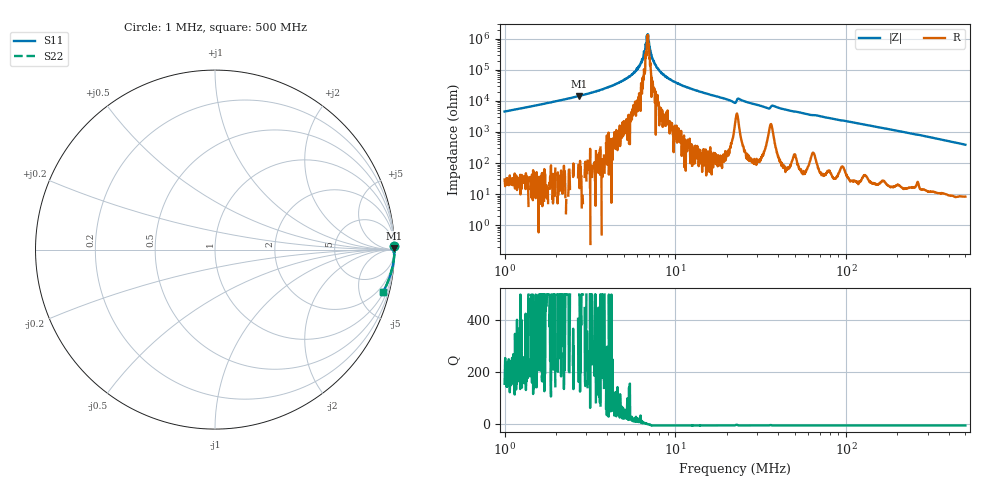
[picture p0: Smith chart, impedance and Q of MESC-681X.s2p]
!s-Parameter Generated by FASTRON Sdn. Bhd.
!FASTRON P/N : MESC-681X
!Keysight Technologies,E4991B,MY54100416,A.01.15
!Date: Fri Mar 27 12:52:29 2026
!Version  : Rev00 Fri Mar 27 12:52:29 2026
!Data & Calibration Information:
!PortZ  Port1:50+j0  Port2:50+j0
!When reading, reference impedance value at option line is always used.
!Remarks : This data is being provided solely for informational purposes.
!Freq	S11	S21	S12	S22
# Hz S dB R 50
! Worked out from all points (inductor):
!   1601 points, 1 MHz to 500 MHz, reference 50 ohm
!   read as one part in series: L = 713 uH near 1.032 MHz
!   highest Q = 942 at 2.745 MHz (marker M1), where L = 849 uH
!   self-resonance near 6.866 MHz
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1000000  -0.00 1.3  -33.22 -88.4  -33.22 -88.4  -0.00 1.3
2745255  -0.00 0.4  -43.31 -89.5  -43.31 -89.5  -0.00 0.4
2820919  -0.00 0.4  -43.64 -89.5  -43.64 -89.5  -0.00 0.4
4257919  -0.00 0.2  -49.74 -89.1  -49.74 -89.1  -0.00 0.2
5502118  -0.00 0.1  -56.67 -86.5  -56.67 -86.5  -0.00 0.1
5900561  -0.00 0.1  -59.62 -87.2  -59.62 -87.2  -0.00 0.1
6206152  -0.00 0.0  -63.32 -86.2  -63.32 -86.2  -0.00 0.0
6451950  -0.00 0.0  -67.45 -82.3  -67.45 -82.3  -0.00 0.0
6707483  -0.00 0.0  -76.90 -69.9  -76.90 -69.9  -0.00 0.0
6892354  -0.00 -0.0  -79.49 7.8  -79.49 7.8  -0.00 -0.0
7027516  -0.00 -0.0  -76.49 58.4  -76.49 58.4  -0.00 -0.0
7449115  -0.00 -0.0  -65.45 81.5  -65.45 81.5  -0.00 -0.0
7957584  -0.00 -0.1  -60.32 84.7  -60.32 84.7  -0.00 -0.1
8941017  -0.00 -0.1  -54.94 86.8  -54.94 86.8  -0.00 -0.1
1.094217e7  -0.00 -0.2  -50.07 89.3  -50.07 89.3  -0.00 -0.2
2.236068e7  -0.02 -0.6  -38.74 77.5  -38.74 77.5  -0.02 -0.6
2.37944e7  -0.01 -0.5  -41.17 83.5  -41.17 83.5  -0.01 -0.5
3.45472e7  -0.01 -1.0  -35.39 83.8  -35.39 83.8  -0.01 -1.0
3.762909e7  -0.01 -0.8  -36.82 83.3  -36.82 83.3  -0.01 -0.8
6.307767e7  -0.02 -1.6  -30.93 85.3  -30.93 85.3  -0.02 -1.6
1.77937e8  -0.04 -4.6  -21.88 84.5  -21.88 84.5  -0.04 -4.6
5e8  -0.32 -14.3  -12.14 74.5  -12.14 74.5  -0.32 -14.3
